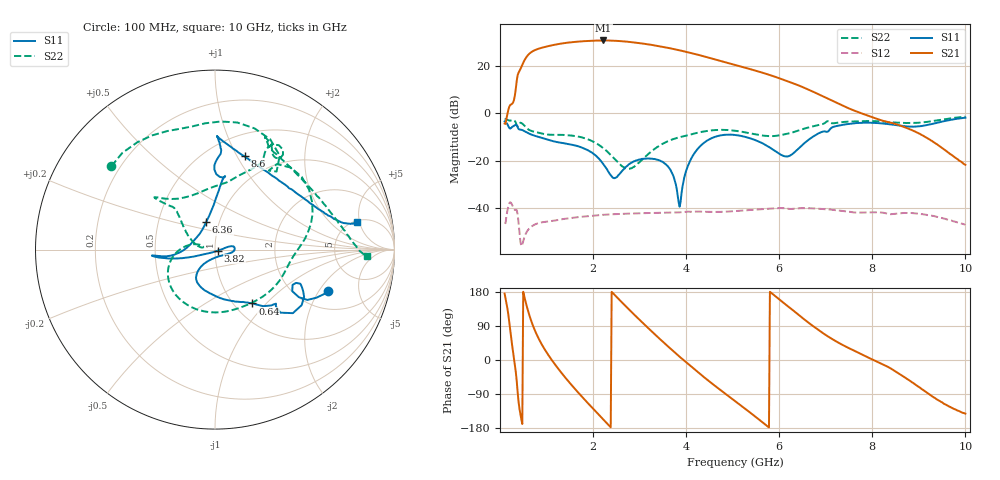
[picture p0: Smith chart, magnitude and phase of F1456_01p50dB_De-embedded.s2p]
! Integrated Device Technology
! Corporate Headquarters
! 6024 Silver Creek Valley Road
! San Jose, CA 95138  USA
! Phone:  1-408-284-8200
! Toll Free:  1-800-223-1366
! Webpage:  http://www.idt.com/
! Timing and RF Division
! 515 Groton Road, Suite 102
! Westford, MA 01886-6024
! Device:  F1456
! Description: 6-bit 0.5 dB Transmit Variable Gain Amplifier
! Frequency:  2100.0 -  2950.00 MHz
! Package:  6x6 mm Thin QFN Plastic Package: 28 pin
! State:  3
! Atten State:  1.5 dB
! Voltage:  +5.00 Volts
! Current:  213.487 mA
! Data:  The device was measured on a the F1455 evaluation board which has
!  individual transmission lines to the RF pins.  Data was collected
!  using a calibrated network analyzer.  The evaluation board was
!  de-embedded using a TRL calibration technique.
!  The reference plane is the edge of the package pin.
!  Pin  1 = CSb
!  Pin  2 = DATA
!  Pin  3 = CLK
!  Pin  4 = RSET
!  Pin  5 = GND
!  Pin  6 = RFIN  = Port 1
!  Pin  7 = GND
!  Pin  8 = NC
!  Pin  9 = NC
!  Pin 10 = NC
!  Pin 11 = NC
!  Pin 12 = NC
!  Pin 13 = NC
!  Pin 14 = /STBY
!  Pin 15 = GND
!  Pin 16 = RFOUT  = Port 2
!  Pin 17 = GND
!  Pin 18 = NC
!  Pin 19 = NC
!  Pin 20 = NC
!  Pin 21 = GND
!  Pin 22 = NC
!  Pin 23 = GND
!  Pin 24 = NC
!  Pin 25 = NC
!  Pin 26 = NC
!  Pin 27 = GND
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# GHz S dB R 50
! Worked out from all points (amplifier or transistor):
!   496 points, 100 MHz to 10 GHz, reference 50 ohm
!   highest |S21| = 30.8 dB at 2.22 GHz (marker M1)
!   |S21| within 3 dB of that: 915.6 MHz to 3.576 GHz (2.661 GHz wide, 118 % of centre)
!   unconditionally stable (mu >= 1): start of sweep to end of sweep
!   at 1.74 GHz: K = 2.19, MAG = 30.9 dB, |S12| = -43.8 dB
!   at 5.06 GHz: K = 4.23, MAG = 21.7 dB, |S12| = -41.4 dB
!   at 10 GHz: K = 139.80, MAG = -11.8 dB, |S12| = -47.1 dB
!   S11 on the Smith chart (normalised r, x): 100 MHz: 2.90, -2.43; 640 MHz: 1.21, -0.84; 3.82 GHz: 1.03, -0.01; 6.36 GHz: 0.87, +0.27; 8.6 GHz: 0.73, +1.08; 10 GHz: 5.24, +4.60
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0.1  -3.47 -20.1  -4.35 175.2  -46.27 41.4  -2.60 141.1
0.34  -4.83 -32.7  10.28 -31.0  -40.87 -143.3  -3.94 55.4
0.42  -6.86 -41.6  17.91 -129.3  -50.63 144.4  -4.13 47.3
0.54  -7.70 -49.8  22.89 159.1  -51.63 -170.2  -5.55 10.7
0.64  -8.74 -55.2  25.35 115.0  -48.52 162.4  -7.18 -5.0
0.84  -10.07 -67.7  27.37 54.4  -46.40 114.6  -8.26 -35.0
1.16  -11.88 -91.6  28.92 -8.0  -45.43 71.6  -9.11 -81.4
1.48  -13.07 -111.4  29.92 -57.6  -44.40 45.2  -9.32 -120.7
1.76  -14.53 -124.3  30.42 -96.7  -43.74 26.5  -10.21 -147.2
2.22  -21.46 -124.4  30.79 -157.0  -42.95 0.1  -14.75 177.0
2.5  -27.14 -57.9  30.63 167.2  -42.65 -14.8  -20.06 162.9
2.84  -20.78 -11.1  30.03 125.1  -42.40 -32.0  -23.12 170.9
3.1  -19.24 -0.1  29.37 94.1  -42.25 -44.4  -18.86 163.5
3.4  -19.76 9.9  28.44 59.5  -42.12 -58.3  -14.06 146.8
3.82  -34.98 -17.0  26.79 13.1  -41.93 -76.7  -10.33 135.0
4.4  -12.26 -168.2  23.97 -46.9  -41.66 -103.7  -7.63 138.8
5.06  -9.19 -174.6  20.36 -109.2  -41.37 -130.3  -7.41 137.3
6.36  -15.93 108.2  12.21 124.8  -40.31 157.0  -7.63 74.3
6.7  -10.24 87.6  9.36 91.9  -40.22 134.3  -5.66 63.4
8.36  -4.62 82.7  -3.80 -19.6  -42.64 62.2  -3.80 62.4
8.6  -5.27 72.4  -5.22 -38.1  -42.29 56.5  -4.04 55.7
10  -1.86 10.9  -21.81 -141.5  -47.11 -20.4  -1.46 -2.5
